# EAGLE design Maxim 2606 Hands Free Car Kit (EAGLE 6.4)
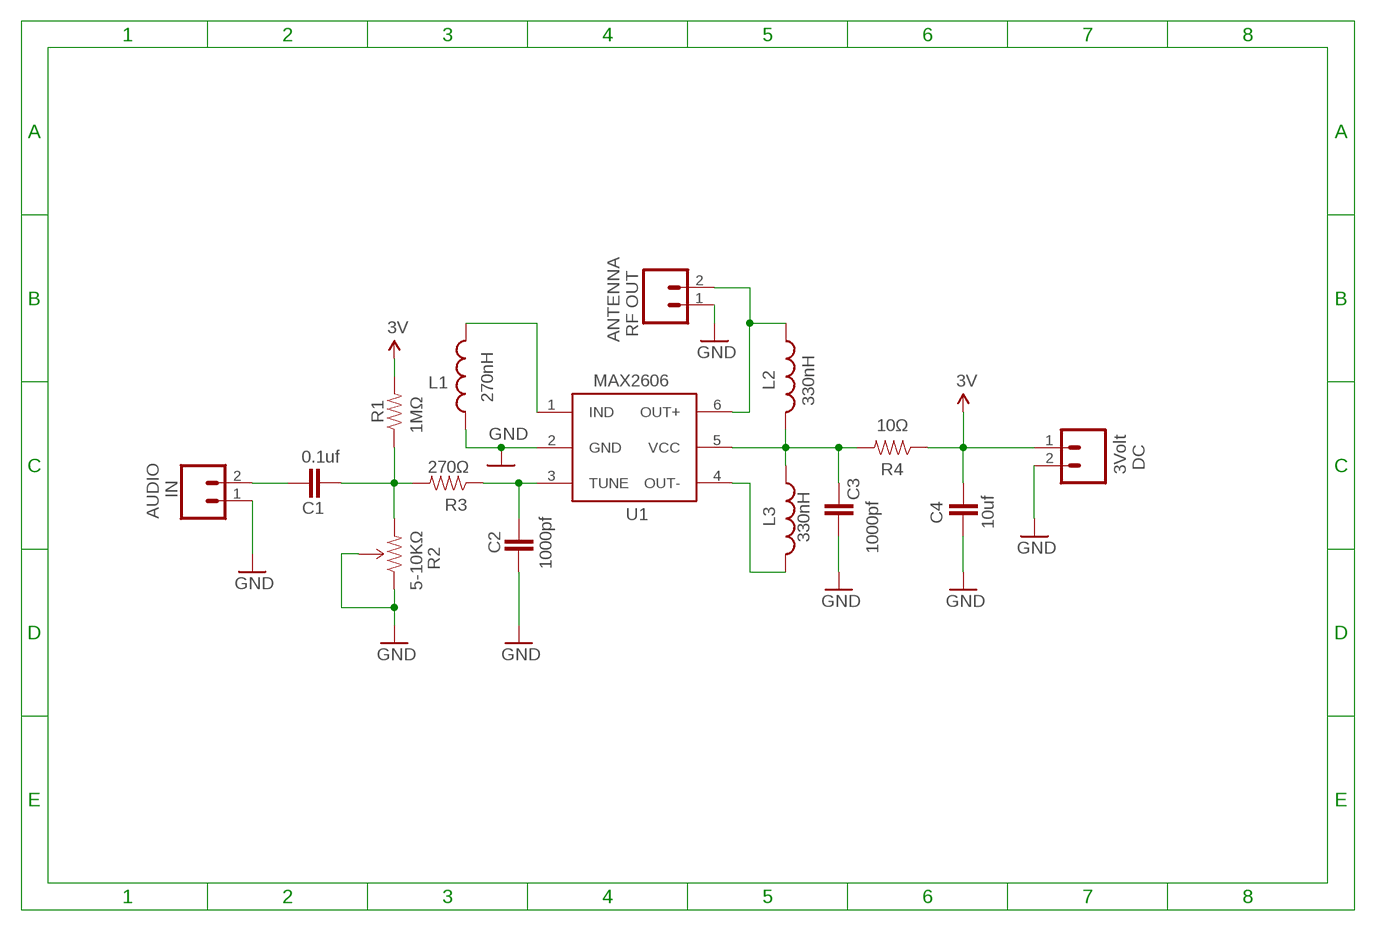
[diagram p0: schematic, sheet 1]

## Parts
ANTENNA  RF OUT  M02PTH  [1X02]
AUDIO  IN  M02PTH  [1X02]
C1  0.1uf  CAP0805  [0805]
C2  1000pf  CAP0805  [0805]
C3  1000pf  CAP0805  [0805]
C4  10uf  CAP0805  [0805]
DC  3Volt  M02PTH  [1X02]
L1  270nH  INDUCTOR0805  [0805]
L2  330nH  INDUCTOR0805  [0805]
L3  330nH  INDUCTOR0805  [0805]
R1  1MΩ  RESISTOR0805-RES  [0805]
R2  5-10KΩ  TRIMPOTSMD  [TRIMPOT-3MM]
R3  270Ω  RESISTOR0805-RES  [0805]
R4  10Ω  RESISTOR0805-RES  [0805]
U1  MAX2606  MAX2606-SOT-23-6L  [MAX2606-SOT-23-6L]

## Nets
GND: ANTENNA.1 AUDIO.1 C2.2 C3.2 C4.2 DC.2 L1.1 R2.1(CCW) R2.2(WIPER) U1.2(GND)
N$1: AUDIO.2 C1.1
N$2: C1.2 R1.1 R2.3(CW) R3.2
N$3: ANTENNA.2 L2.1 U1.6(OUT+)
N$4: C2.1 R3.1 U1.3(TUNE)
N$5: L1.2 U1.1(IND)
N$6: L3.2 U1.4(OUT-)
N$7: C3.1 L2.2 L3.1 R4.2 U1.5(VCC)
VCC: C4.1 DC.1 R1.2 R4.1 ; supply symbol labelled 3V

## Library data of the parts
ANTENNA AUDIO DC = SparkFun-Connectors:M02: Standard 2-pin 0.1" header. Use with
C1-C4 = SparkFun-Capacitors:CAP: Capacitor
L1-L3 = SparkFun-Passives:INDUCTOR: Inductors
R1 R3 R4 = SparkFun-Resistors:RESISTOR: Resistor
R2 = SparkFun-Electromechanical:TRIMPOT: Various small potentiometers for "set-and-forget" applications
U1 = MAX2606:MAX2606-SOT-23-6L

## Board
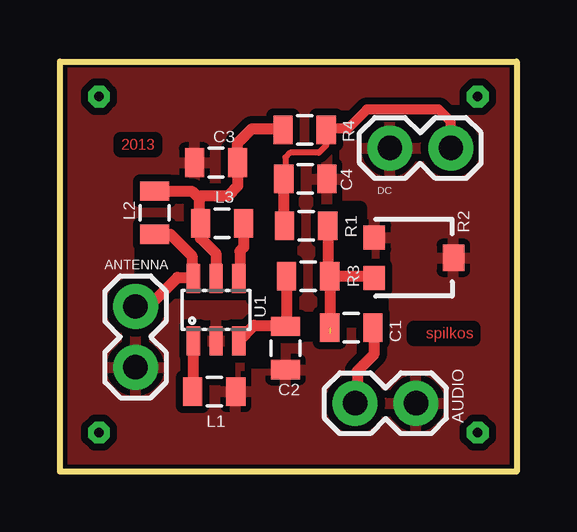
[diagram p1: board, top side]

Size 19.06 x 17.17 mm. Coordinates in mm from the lower left corner, seen from the top.
Outline: 0,0 19.06,0 19.06,17.17 0,17.17 0,0
Copper layers (1*16): Top 0.035mm / dielectric 1.5mm / Bottom 0.035mm
Design rules "SparkFun": minimum track width 8mil, minimum drill 20mil, track to track 8mil, track to pad 8mil, pad to pad 8mil, via to via 8mil, smd to smd 8mil, copper to edge 10mil, drill to drill 8mil, minimum pad ring 12mil, minimum via ring 10mil, stop-mask expansion 4mil, vias tented up to drill 25mil, thermal gap 10mil
tRestrict: area 11.2,6.3 to 13.4,7.5; area 6,3.9 to 7,4.7; area 8,4.6 to 8.9,5.5; area 8.1,7.2 to 9.1,9.1; area 11.7,8.7 to 12.7,9.5; area 11.8,9.8 to 12.5,11; area 3.4,8 to 4.8,9.2
Milling: 4 lines

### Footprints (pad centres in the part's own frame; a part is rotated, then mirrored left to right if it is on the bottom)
1X02 = drill 1.016 pad 1.88: 1 0,0; 2 2.54,0
0805 = smd 0.8 x 1.2: 1 -0.9,0; 2 0.9,0
TRIMPOT-3MM = smd 1 x 0.9: 1 -0.85,-1.65; 3 0.85,-1.65 | smd 1.1 x 0.9: 2 0,1.65
MAX2606-SOT-23-6L = smd 1.2 x 0.55: 1 -1.3,0.95; 2 -1.3,0; 3 -1.3,-0.95; 4 1.3,-0.95; 5 1.3,0; 6 1.3,0.95

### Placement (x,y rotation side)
ANTENNA  3.15,4.35 90 top
AUDIO  14.85,2.85 180 top
C1  12.15,6 180 top
C2  9.41,5.15 270 top
C3  6.51,12.89 180 top
C4  10.23,12.21 0 top
DC  16.3,13.5 180 top
L1  6.43,3.34 180 top
L2  3.95,10.8 90 top
L3  6.76,10.36 0 top
R1  10.27,10.25 180 top
R2  14.76,8.92 270 top
R3  10.35,8.15 0 top
R4  10.2,14.25 180 top
U1  6.51,6.75 90 top

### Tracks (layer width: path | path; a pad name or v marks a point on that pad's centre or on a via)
GND
  pour Top (isolate 0.305): 0,17.2 18.7,17.2 18.7,0 0,0
N$1
  Top 0.406: 13.11,5.94 C1.1
  Top 0.457: AUDIO.2 12.4,2.94 12.4,4.2 13.11,4.91 13.11,5.94
N$2  (1 unrouted)
  Top 0.457: R3.2 11.25,5.76 | R3.2 13.03,8.15 R2.3 | R1.1 11.17,8.23 R3.2
N$3
  Top 0.457: L2.1 4.6,9.9 5.5,9 5.5,8.11 U1.6 5.51,8.1 4.9,8.1 3.69,6.89 ANTENNA.2
N$4
  Top 0.457: U1.3 8.1,6.1 9.36,6.1 C2.1 9.45,6.09 R3.1
N$5
  Top 0.457: U1.1 5.56,3.37 L1.2
N$6
  Top 0.457: L3.2 7.66,9.36 7.5,9.2 7.5,8.09 U1.4
N$7
  Top 0.457: U1.5 6.5,9.1 5.86,9.74 L3.1 5.8,10.42 5.8,11.4 | L2.2 5.5,11.7 5.8,11.4 | 5.8,11.4 5.9,11.5 7,11.5 7.41,11.91 C3.1 7.41,13.71 8,14.3 9.25,14.3 R4.2
N$8  (via drill 0.4 pad 0.35)
  other vias: 1.63,15.64
N$9  (via drill 0.4 pad 0.35)
  other vias: 1.63,1.63
N$10  (via drill 0.4 pad 0.35)
  other vias: 17.42,1.63
N$11  (via drill 0.4 pad 0.35)
  other vias: 17.42,15.64
VCC
  Top 0.254: R4.1 11.1,13.6 10.8,13.3 9.6,13.3 9.4,13.1 9.4,12.28 C4.1
  Top 0.406: DC.1 16.3,14.6 15.8,15.1 12.8,15.1 12,14.3 11.15,14.3 R4.1
  Top 0.457: C4.1 9.33,10.29 R1.2 | 11.15,14.2 R4.1

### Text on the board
Top: 2013 | spilkos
